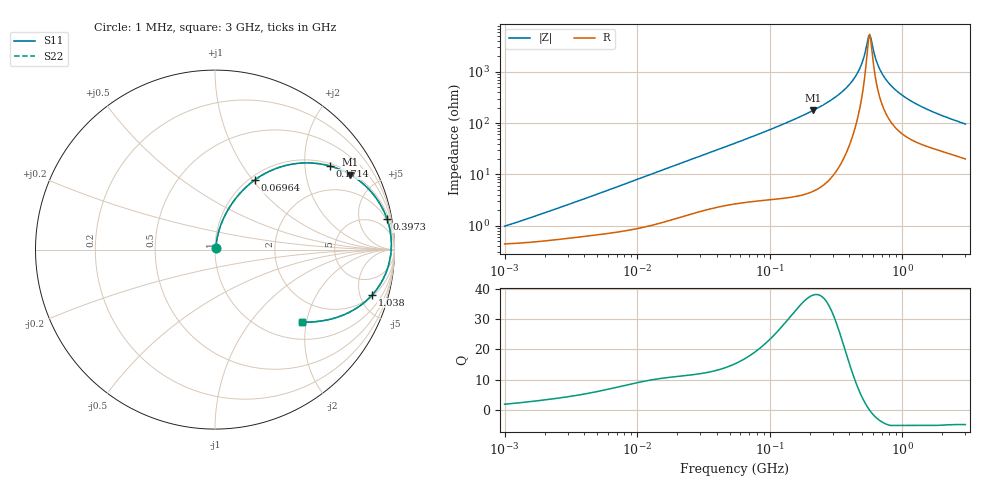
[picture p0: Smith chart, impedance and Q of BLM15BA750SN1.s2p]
! BLM15BA750SN1
# Hz S RI R 50
!Freq.(Hz) S11(Real) S11(Imag) S21(Real) S21(Imag) S12(Real) S12(Imag) S22(Real) S22(Imag)
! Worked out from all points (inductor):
!   401 points, 1 MHz to 3 GHz, reference 50 ohm
!   read as one part in series: L = 135 nH near 1.717 MHz
!   highest Q = 37.9 at 213.6 MHz (marker M1), where L = 132 nH
!   self-resonance near 558.4 MHz
!   S11 on the Smith chart (normalised r, x): 1 MHz: 1.01, +0.02; 69.64 MHz: 1.06, +1.03; 171.4 MHz: 1.08, +2.69; 397.3 MHz: 2, +11; 1.038 GHz: 2.15, -6.43; 3 GHz: 1.40, -1.88
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1000000  0.00445 0.00863  0.9955 -0.00863  0.9955 -0.00863  0.00445 0.00863
3823119  0.00701 0.0311  0.993 -0.0311  0.993 -0.0311  0.00701 0.0311
1.461624e7  0.0234 0.1105  0.9766 -0.1105  0.9766 -0.1105  0.0234 0.1105
5.477226e7  0.1569 0.3324  0.8431 -0.3324  0.8431 -0.3324  0.1569 0.3324
6.964249e7  0.2216 0.3881  0.7784 -0.3881  0.7784 -0.3881  0.2216 0.3881
1.148668e8  0.4276 0.4758  0.5724 -0.4758  0.5724 -0.4758  0.4276 0.4758
1.714156e8  0.6411 0.4655  0.3589 -0.4655  0.3589 -0.4655  0.6411 0.4655
2.094008e8  0.7441 0.4233  0.2559 -0.4233  0.2559 -0.4233  0.7441 0.4233
2.136344e8  0.7538 0.4178  0.2462 -0.4178  0.2462 -0.4178  0.7538 0.4178
3.062963e8  0.8974 0.2876  0.1026 -0.2876  0.1026 -0.2876  0.8974 0.2876
3.973271e8  0.9585 0.1701  0.0415 -0.1701  0.0415 -0.1701  0.9585 0.1701
4.75755e8  0.9788 0.0845  0.0212 -0.0845  0.0212 -0.0845  0.9788 0.0845
5.051982e8  0.9817 0.0558  0.0183 -0.0558  0.0183 -0.0558  0.9817 0.0558
5.473095e8  0.9825 0.0178  0.0175 -0.0178  0.0175 -0.0178  0.9825 0.0178
5.696638e8  0.9817 -0.000997  0.0183 0.000997  0.0183 0.000997  0.9817 -0.000997
5.81181e8  0.981 -0.0104  0.019 0.0104  0.019 0.0104  0.981 -0.0104
6.296259e8  0.9761 -0.0474  0.0239 0.0474  0.0239 0.0474  0.9761 -0.0474
6.685918e8  0.9703 -0.0747  0.0297 0.0747  0.0297 0.0747  0.9703 -0.0747
8.005644e8  0.9424 -0.1527  0.0576 0.1527  0.0576 0.1527  0.9424 -0.1527
1.038491e9  0.8773 -0.2508  0.1227 0.2508  0.1227 0.2508  0.8773 -0.2508
1.613037e9  0.7212 -0.3619  0.2788 0.3619  0.2788 0.3619  0.7212 -0.3619
3e9  0.4829 -0.4046  0.5171 0.4046  0.5171 0.4046  0.4829 -0.4046
